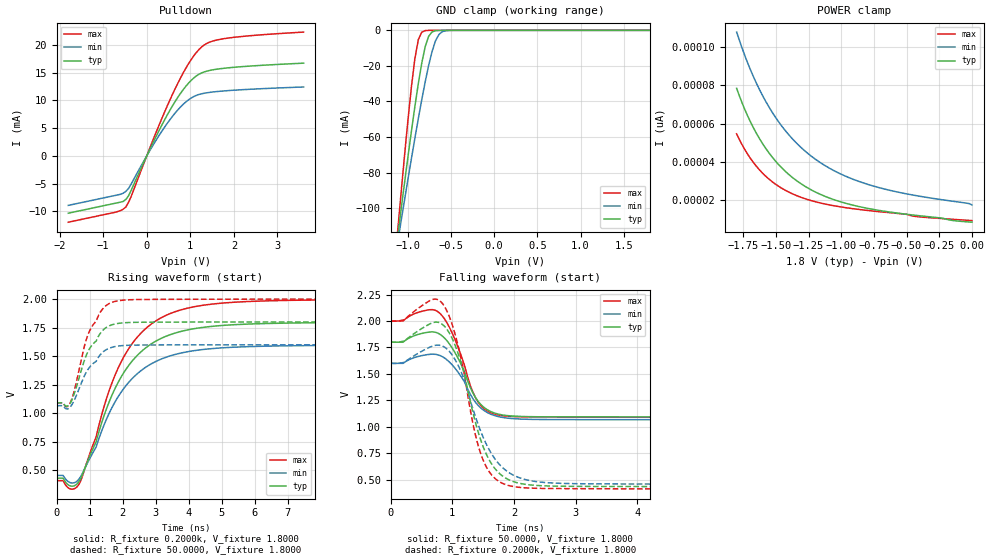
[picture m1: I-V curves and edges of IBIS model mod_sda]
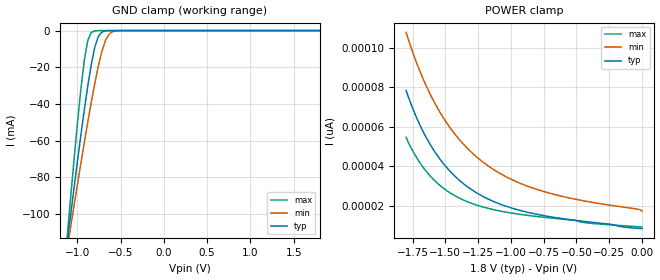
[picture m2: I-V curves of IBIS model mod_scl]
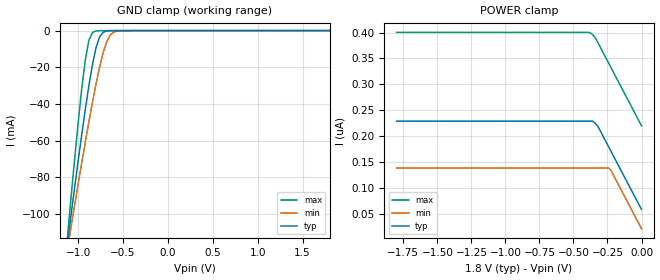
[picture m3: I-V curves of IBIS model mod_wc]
| IBIS (I/O, Buffer, Information, Specification) Model, officially
| electronic behavioral standard for Buffer structures of digital pins.
[IBIS ver]  4.0
[File name] m24512e_1d8_dfn8.ibs
[File Rev]  1.0
[Date]   26 Jan 2023
[Source]   CAD & Design Services (Catania) - STMicroelectronics
[Notes]
   (Note1)  This IBIS model includes the DFN8 package parasitic data
   (Note2)  This IBIS model has some Notes about the non-monotonicity
   of the I-V curves, but they are not indicative of problems
   inside the model;
[Disclaimer]
   Customers are solely responsible for all aspects of their
   own product designs or applications using this IBIS Model.
   STMicroelectronics assumes no liability for Custmer Designs
   and applications associated to this IBIS Model.
   In the use of this IBIS Model Customer shall not modify,
   disassemble, alter this Model in whole or in part.
   If Customers do not accept these terms, the IBIS Model
   may not be used. For any problems or modifications please
   contact STMicroelectronics (www.st.com).
[Copyright] (c) 2023 STMicroelectronics
|   Component M24512E
[Component] M24512E
[Manufacturer] STMicroelectronics
[Package]
| variable  typ   min   max
R_pkg   0.0   0.0   0.0
L_pkg   0.0H   0.0H   0.0H
C_pkg   0.0F   0.0F   0.0F
[Pin]   signal_name   model_name   R_pin   L_pin   C_pin
1   NC   NC   0.0   0.0   0.0
2   NC   NC   0.0   0.0   0.0
3   NC   NC   0.0   0.0   0.0
4   VSS   GND   0.0   0.0   0.0
5   SDA   mod_sda   0.0   0.0   0.0
6   SCL   mod_scl   0.0   0.0   0.0
7   WC   mod_wc   0.0   0.0   0.0
8   VCC   POWER   0.0   0.0   0.0
[Package Model]  182694_DFN8   | also called 182694_MLP_2x3
[Define Package Model]  182694_DFN8
[Manufacturer]  STMicroelectronics
[OEM]  STMicroelectronics
[Description]  8 pin DFN8 2x3
[Number Of Pins]  8
[Pin Numbers]
|Pin Num   Terminal Name
1   | net1
2   | net2
3   | net3
4   | net4_GND
5   | net5
6   | net6
7   | net7
8   | net8_VDD
[Model Data]
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[End Model Data]
[End Package Model]
| Models and submodels in the file (3): mod_sda (I/O_open_drain), mod_scl (Input), mod_wc (Input)
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|   Model mod_sda
[Model]   mod_sda
Model_type I/O_open_drain
Polarity   Inverting
Enable   Active-High
Vinl   =   0.450V
Vinh   =   1.350V
Vmeas  =   0.900V
Cref   =   30pF
Rref   =   500
Vref   =   1.800V
C_comp   2.547pF   2.323pF   2.667pF
[Model Spec]
Vinl   0.450V  0.400V  0.500V  | <- for Vcc = 1.8V, 1.6V, 2.0V
Vinh   1.350V  1.200V  1.500V  | <- for Vcc = 1.8V, 1.6V, 2.0V
Vmeas  0.900V  0.800V  1.000V  | <- for Vcc = 1.8V, 1.6V, 2.0V
[Temperature Range]  25.0000   85.0000   -40.0000
[Voltage Range]   1.8000V   1.6000V   2.0000V
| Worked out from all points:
|   slope of the pulldown table from 0 to 0.27 V, typ, clamps not added: 61.5 ohm
|   GND clamp passes 1 mA (typ) near -0.72 V on its own axis
|   rising waveform, R_fixture 0.2000k, V_fixture 1.8000: 20-80 % time 1.38ns typ, 1.38ns min, 1.37ns max; typ from 0.433 V to 1.8 V
|   rising waveform, R_fixture 50.0000, V_fixture 1.8000: 20-80 % time 635ps typ, 648ps min, 615ps max; typ from 1.09 V to 1.8 V
|   falling waveform, R_fixture 50.0000, V_fixture 1.8000: 20-80 % time 345ps typ, 350ps min, 331ps max; typ from 1.8 V to 1.09 V
|   falling waveform, R_fixture 0.2000k, V_fixture 1.8000: 20-80 % time 400ps typ, 475ps min, 345ps max; typ from 1.8 V to 0.433 V
[Pulldown]
|Voltage   I(typ)   I(min)   I(max)
-1.8V     -10.34mA   -8.93mA    -11.96mA
-720mV    -8.54mA    -7.13mA    -10.16mA
-480mV    -7.859mA   -6.398mA   -9.229mA
-360mV    -6.255mA   -5.118mA   -7.377mA
240mV     3.924mA    3.151mA    4.736mA
600mV     9.149mA    7.235mA    11.26mA
960mV     13.14mA    10.13mA    16.65mA
1.14V     14.44mA    10.93mA    18.68mA
1.26V     14.98mA    11.21mA    19.66mA
1.5V      15.51mA    11.52mA    20.69mA
1.86V     15.88mA    11.78mA    21.26mA
3.6V      16.73mA    12.44mA    22.34mA
[GND_clamp]
|Voltage   I(typ)   I(min)   I(max)
-1.8V     -389.2mA   -332.1mA   -507.3mA
-1.12V    -116.3mA   -119.5mA   -113.3mA
-1.08V    -101mA     -107.4mA   -91.66mA
-1V       -71.13mA   -83.74mA   -50.44mA
-920mV    -42.94mA   -60.76mA   -15.96mA
-880mV    -29.99mA   -49.68mA   -5.261mA
-840mV    -18.43mA   -39.01mA   -1.028mA
-800mV    -9.166mA   -28.93mA   -159.1uA
-760mV    -3.325mA   -19.7mA    -26.96uA
-680mV    -202.6uA   -5.819mA   -1.339uA
-600mV    -10.23uA   -725.2uA   -32.48nA
1.8V      8.512pA    19.96pA    8.401pA
[POWER_clamp]
|Voltage   I(typ)   I(min)   I(max)
-1.8V     78.43pA    107.8pA    54.66pA
-1.74V    67.81pA    96.01pA    46.75pA
-1.68V    58.96pA    85.83pA    40.47pA
-1.62V    51.57pA    77.07pA    35.46pA
-1.54V    43.56pA    67.25pA    30.3pA
-1.46V    37.24pA    59.19pA    26.45pA
-1.38V    32.23pA    52.55pA    23.54pA
-1.2V     24.35pA    41.52pA    19.23pA
-1V       19.06pA    33.56pA    16.45pA
-760mV    15.25pA    27.51pA    14.36pA
-500mV    12.65pA    23.3pA     12.6pA
0V        8.512pA    17.5pA     9.335pA
[Ramp]
| variable   typ   min   max
dV/dt_r   0.3503/0.4041n   0.2673/0.4372n   0.4511/0.3936n
dV/dt_f   0.3503/0.3740n   0.2672/0.3732n   0.4511/0.3823n
R_load = 50.0000
[Rising Waveform]
R_fixture= 0.2000k
V_fixture= 1.8000
V_fixture_min= 1.6000
V_fixture_max= 2.0000
|time   V(typ)   V(min)   V(max)
0s        432.5mV    456.4mV    411.1mV
430ps     363.6mV    391.8mV    337.5mV
660ps     394.8mV    417.4mV    370mV
1.2ns     750.6mV    704.6mV    794.2mV
1.58ns    1.09V      991.6mV    1.187V
1.92ns    1.299V     1.169V     1.428V
2.48ns    1.517V     1.355V     1.678V
3.16ns    1.654V     1.473V     1.835V
5.08ns    1.77V      1.574V     1.966V
10ns      1.796V     1.597V     1.996V
[Rising Waveform]
R_fixture= 50.0000
V_fixture= 1.8000
V_fixture_min= 1.6000
V_fixture_max= 2.0000
|time   V(typ)   V(min)   V(max)
0s        1.092V     1.067V     1.091V
200ps     1.092V     1.067V     1.091V
310ps     1.062V     1.038V     1.058V
400ps     1.082V     1.05V      1.082V
540ps     1.174V     1.116V     1.201V
840ps     1.461V     1.325V     1.582V
980ps     1.555V     1.396V     1.707V
1.38ns    1.72V      1.53V      1.908V
1.72ns    1.778V     1.581V     1.975V
10ns      1.8V       1.6V       2V
[Falling Waveform]
R_fixture= 50.0000
V_fixture= 1.8000
V_fixture_min= 1.6000
V_fixture_max= 2.0000
|time   V(typ)   V(min)   V(max)
0s        1.8V       1.6V       2V
200ps     1.8V       1.6V       2V
610ps     1.895V     1.684V     2.105V
790ps     1.878V     1.676V     2.077V
1.03ns    1.714V     1.564V     1.844V
1.29ns    1.374V     1.31V      1.394V
1.39ns    1.264V     1.222V     1.261V
1.55ns    1.168V     1.141V     1.155V
1.77ns    1.117V     1.094V     1.109V
10ns      1.093V     1.067V     1.091V
[Falling Waveform]
R_fixture= 0.2000k
V_fixture= 1.8000
V_fixture_min= 1.6000
V_fixture_max= 2.0000
|time   V(typ)   V(min)   V(max)
0s        1.8V       1.6V       2V
680ps     1.984V     1.764V     2.204V
860ps     1.958V     1.758V     2.149V
1.08ns    1.717V     1.597V     1.798V
1.34ns    1.122V     1.158V     1.015V
1.46ns    877.5mV    958.6mV    748.4mV
1.64ns    647.4mV    742.2mV    544.7mV
1.9ns     505.1mV    575.4mV    448.3mV
2.82ns    439.1mV    465.7mV    416.8mV
10ns      433.2mV    457.2mV    411.6mV
|   Model mod_scl
[Model]   mod_scl
Model_type Input
Vinl   =   0.450V
Vinh   =   1.350V
C_comp   1.062pF   1.014pF   1.112pF
[Model Spec]
Vinl   0.450V  0.400V  0.500V  | <- for Vcc = 1.8V, 1.6V, 2.0V
Vinh   1.350V  1.200V  1.500V  | <- for Vcc = 1.8V, 1.6V, 2.0V
[Temperature Range]  25.0000   85.0000   -40.0000
[Voltage Range]   1.8000V   1.6000V   2.0000V
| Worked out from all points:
|   GND clamp passes 1 mA (typ) near -0.72 V on its own axis
[GND_clamp]
|Voltage   I(typ)   I(min)   I(max)
-1.8V     -389.2mA   -332.1mA   -507.3mA
-1.12V    -116.3mA   -119.5mA   -113.3mA
-1.08V    -101mA     -107.4mA   -91.66mA
-1V       -71.13mA   -83.74mA   -50.44mA
-920mV    -42.94mA   -60.76mA   -15.96mA
-880mV    -29.99mA   -49.68mA   -5.261mA
-840mV    -18.43mA   -39.01mA   -1.028mA
-800mV    -9.166mA   -28.93mA   -159.1uA
-760mV    -3.325mA   -19.7mA    -26.96uA
-680mV    -202.6uA   -5.819mA   -1.339uA
-600mV    -10.23uA   -725.2uA   -32.48nA
1.8V      8.512pA    19.96pA    8.401pA
[POWER_clamp]
|Voltage   I(typ)   I(min)   I(max)
-1.8V     78.43pA    107.8pA    54.66pA
-1.74V    67.81pA    96.01pA    46.75pA
-1.68V    58.96pA    85.83pA    40.47pA
-1.62V    51.57pA    77.07pA    35.46pA
-1.54V    43.56pA    67.25pA    30.3pA
-1.46V    37.24pA    59.19pA    26.45pA
-1.38V    32.23pA    52.55pA    23.54pA
-1.2V     24.35pA    41.52pA    19.23pA
-1V       19.06pA    33.56pA    16.45pA
-760mV    15.25pA    27.51pA    14.36pA
-500mV    12.65pA    23.3pA     12.6pA
0V        8.512pA    17.5pA     9.335pA
|   Model mod_wc
[Model]   mod_wc
Model_type Input
Vinl   =   0.450V
Vinh   =   1.350V
C_comp   1.062pF   1.014pF   1.112pF
[Model Spec]
Vinl   0.450V  0.400V  0.500V  | <- for Vcc = 1.8V, 1.6V, 2.0V
Vinh   1.350V  1.200V  1.500V  | <- for Vcc = 1.8V, 1.6V, 2.0V
[Temperature Range]  25.0000   85.0000   -40.0000
[Voltage Range]   1.8000V   1.6000V   2.0000V
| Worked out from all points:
|   GND clamp passes 1 mA (typ) near -0.72 V on its own axis
[GND_clamp]
|Voltage   I(typ)   I(min)   I(max)
-1.8V     -389.2mA   -332.1mA   -507.3mA
-1.12V    -116.3mA   -119.5mA   -113.3mA
-1.08V    -101mA     -107.5mA   -91.66mA
-1V       -71.13mA   -83.75mA   -50.44mA
-920mV    -42.94mA   -60.76mA   -15.97mA
-880mV    -29.99mA   -49.68mA   -5.268mA
-840mV    -18.43mA   -39.01mA   -1.039mA
-800mV    -9.17mA    -28.93mA   -171.5uA
-760mV    -3.331mA   -19.7mA    -40.56uA
-680mV    -212.1uA   -5.822mA   -15.24uA
-600mV    -20.7uA    -731.4uA   -11.33uA
1.8V      17.12uA    16.16uA    18.32uA
[POWER_clamp]
|Voltage   I(typ)   I(min)   I(max)
-1.8V     229.3nA    138.9nA    400.3nA
-380mV    229.3nA    138.9nA    400nA
-360mV    229.3nA    138.9nA    396.2nA
-340mV    225.2nA    138.9nA    390nA
-320mV    219nA      138.9nA    380.3nA
-240mV    179nA      138.9nA    340.3nA
-220mV    169nA      132.1nA    330.3nA
0V        59nA       22nA       220.3nA
